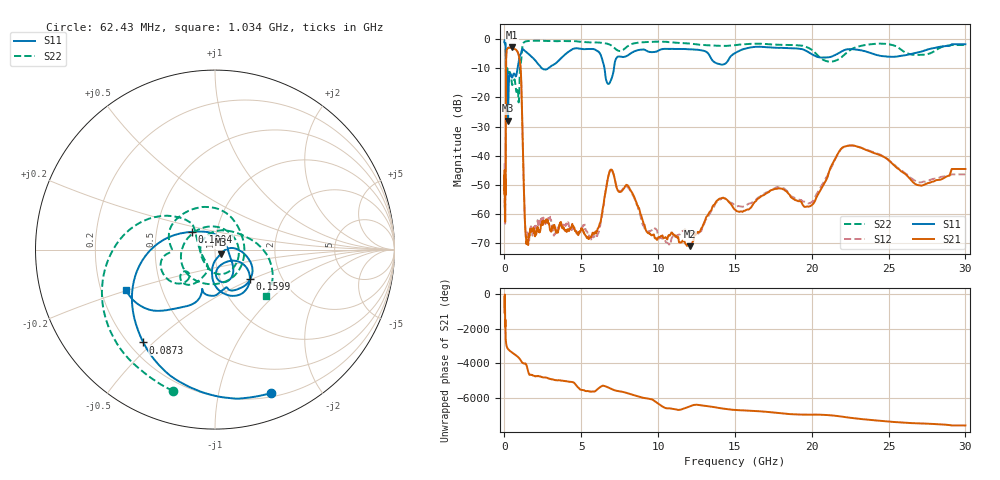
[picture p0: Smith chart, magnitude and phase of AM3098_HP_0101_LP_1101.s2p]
! Date/Time: Thu, Feb 28, 2019 8:36 AM
! Network Analyzer: Agilent Technologies E8364B Rev: A.07.50.67
! Sweep from 0.010 to 30.000 GHz, 1601 Points, Sweep Type: LOG
! Power Supply: 5.022 V, 0.002 A
# Hz S DB R 50
!freq MagS11 AngS11 MagS21 AngS21 MagS12 AngS12 MagS22 AngS22
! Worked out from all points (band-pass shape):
!   1601 points, 10 MHz to 30 GHz, reference 50 ohm
!   highest |S21| = -2.79 dB at 493.1 MHz (marker M1); lowest = -71.2 dB at 12.07 GHz (marker M2)
!   |S21| within 3 dB of the highest: 114.6 MHz to 945 MHz (830.4 MHz wide, 157 % of centre)
!   lowest |S11| = -28.0 dB at 236.3 MHz (marker M3), VSWR 1.08, Z = 53.1 - j2.72 ohm
!   |S11| at or under -10 dB: 97.47 MHz to 849.7 MHz (752.3 MHz wide, 159 % of centre); 2.458 GHz to 2.834 GHz (376.1 MHz wide, 14.2 % of centre); 6.511 GHz to 7.124 GHz (613.3 MHz wide, 9 % of centre)
!   |S22| runs from -22.2 to -0.4 dB; largest |S21 - S12| = 0.012
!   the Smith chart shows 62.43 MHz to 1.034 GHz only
!   S11 on the Smith chart (normalised r, x): 62.43 MHz: 0.23, -1.44; 87.3 MHz: 0.26, -0.46; 100.4 MHz: 0.76, +0.16; 159.9 MHz: 1.38, -0.48; 1.034 GHz: 0.31, -0.20
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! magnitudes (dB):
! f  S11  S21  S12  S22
! 10 MHz  -0.4  -47.0  -43.0  -0.6
! 38.04 MHz  -0.5  -58.6  -61.7  -1.0
! 62.43 MHz  -1.3  -50.6  -52.3  -1.7
! 87.3 MHz  -3.7  -39.5  -39.1  -4.1
! 100.4 MHz  -15.8  -13.3  -13.3  -20.1
! 144.7 MHz  -17.5  -3.7  -3.7  -13.7
! 159.9 MHz  -11.9  -3.5  -3.5  -11.1
! 236.3 MHz  -28.0  -2.9  -2.9  -12.1
! 493.1 MHz  -13.2  -2.8  -2.8  -15.6
! 550.5 MHz  -12.4  -3.0  -3.0  -15.0
! 926.3 MHz  -7.8  -5.4  -5.3  -21.7
! 1.034 GHz  -5.3  -8.9  -8.8  -8.3
! 1.389 GHz  -4.2  -68.1  -67.2  -0.7
! 2.084 GHz  -7.7  -66.7  -64.9  -0.5
! 5.812 GHz  -3.4  -67.0  -67.7  -1.0
! 6.855 GHz  -14.9  -45.3  -45.3  -1.8
! 7.926 GHz  -5.8  -50.1  -50.6  -2.7
! 12.07 GHz  -3.4  -71.2  -66.6  -1.4
! 14.09 GHz  -8.7  -54.8  -55.0  -2.3
! 19.8 GHz  -4.5  -57.6  -56.5  -3.0
! 22.56 GHz  -3.3  -36.5  -36.6  -3.5
! 30 GHz  -1.7  -44.6  -46.5  -1.9
